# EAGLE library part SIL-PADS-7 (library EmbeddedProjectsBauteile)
Anschlüsse 2,54mm Raster, SMT oder THT
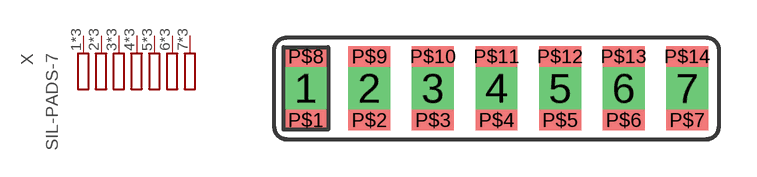
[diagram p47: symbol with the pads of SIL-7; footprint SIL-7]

Designator prefix X

## SIL-PADS-7  [SIL-7]
1  1  pas
2  2  pas
3  3  pas
4  4  pas
5  5  pas
6  6  pas
7  7  pas
P$1  1  pas
P$2  2  pas
P$3  3  pas
P$4  4  pas
P$5  5  pas
P$6  6  pas
P$7  7  pas
P$8  1  pas
P$9  2  pas
P$10  3  pas
P$11  4  pas
P$12  5  pas
P$13  6  pas
P$14  7  pas

## Footprint SIL-7 (pad centres in mm)
drill 0.813 pad 1.676 square: 1 0,0; 2 2.54,0; 3 5.08,0; 4 7.62,0; 5 10.16,0; 6 12.7,0; 7 15.24,0
smd 1.676 x 0.813: P$1 0,-1.27; P$2 2.54,-1.27; P$3 5.08,-1.27; P$4 7.62,-1.27; P$5 10.16,-1.27; P$6 12.7,-1.27; P$7 15.24,-1.27; P$8 0,1.27; P$9 2.54,1.27; P$10 5.08,1.27; P$11 7.62,1.27; P$12 10.16,1.27; P$13 12.7,1.27; P$14 15.24,1.27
